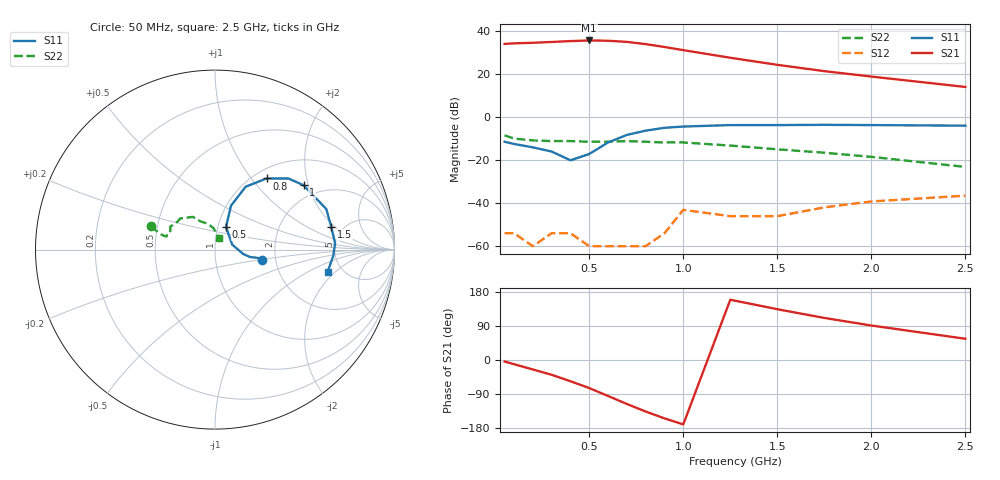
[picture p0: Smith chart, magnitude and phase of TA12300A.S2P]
!  ITA-06300  S-PARAMETERS
!  VCC - Vee =5 V  LAST UPDATED 07-22-92
# ghz s ma r 50
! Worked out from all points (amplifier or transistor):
!   16 points, 50 MHz to 2.5 GHz, reference 50 ohm
!   highest |S21| = 35.8 dB at 500 MHz (marker M1)
!   |S21| within 3 dB of that: start of sweep to 897.3 MHz
!   unconditionally stable (mu >= 1): start of sweep to end of sweep
!   at 200 MHz: K = 8.04, MAG = 35.3 dB, |S12| = -60.0 dB
!   at 800 MHz: K = 7.05, MAG = 35.6 dB, |S12| = -60.0 dB
!   at 2.5 GHz: K = 3.90, MAG = 16.5 dB, |S12| = -36.5 dB
!   S11 on the Smith chart (normalised r, x): 50 MHz: 1.70, -0.21; 500 MHz: 1.09, +0.28; 800 MHz: 1.14, +1.19; 1 GHz: 1.63, +1.86; 1.5 GHz: 4.04, +1.80; 2.5 GHz: 3.86, -1.60
0.05  0.27 -12.0  51.3 -4.0  0.002 -89.0  0.38 160.0
0.1  0.24 -11.0  52.8 -11.0  0.002 -51.0  0.32 164.0
0.2  0.2 -12.0  54.5 -25.0  0.001 -158.0  0.29 165.0
0.3  0.16 -9.0  56.9 -39.0  0.002 20.0  0.28 165.0
0.4  0.1 16.0  59.6 -56.0  0.002 35.0  0.28 162.0
0.5  0.14 64.0  61.7 -74.0  0.001 109.0  0.27 160.0
0.6  0.26 70.0  60.7 -95.0  0.001 16.0  0.27 157.0
0.7  0.39 64.0  57.2 -116.0  0.001 -40.0  0.28 153.0
0.8  0.49 54.0  50.7 -136.0  0.001 -150.0  0.27 148.0
0.9  0.57 44.0  43.5 -154.0  0.002 90.0  0.26 143.0
1  0.61 36.0  36.7 -170.0  0.007 93.0  0.26 138.1
1.25  0.66 20.0  24.4 159.0  0.005 138.0  0.22 124.0
1.5  0.66 11.0  16.7 134.0  0.005 107.0  0.18 118.0
1.75  0.67 3.0  11.9 111.0  0.008 103.0  0.15 106.0
2  0.66 -3.0  8.9 91.0  0.011 115.0  0.12 94.0
2.5  0.64 -11.0  5.1 56.0  0.015 126.0  0.07 71.0
